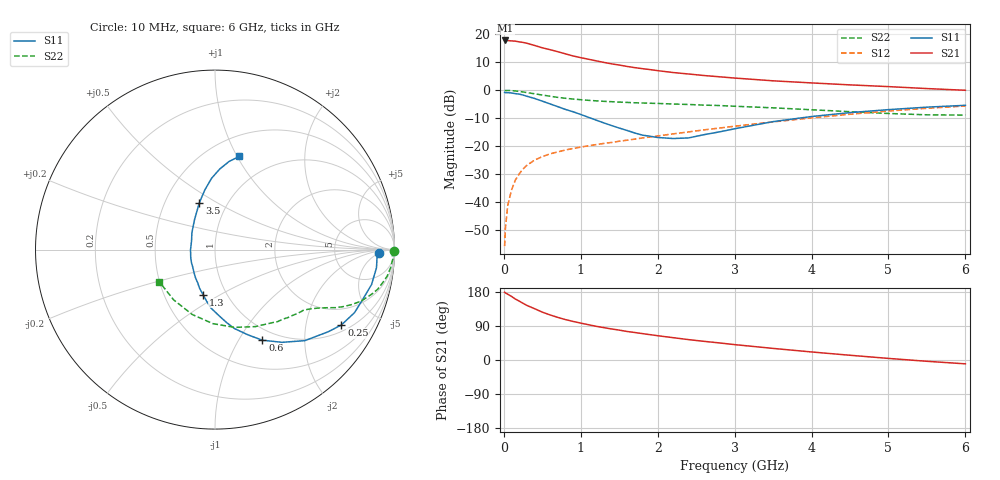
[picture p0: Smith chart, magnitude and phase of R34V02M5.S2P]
! SIEMENS Small Signal Semiconductors
! BFR181
! Si NPN RF Bipolar Junction Transistor in SOT23
! VCE = 4 V  IC = 2.5 mA
! Common Emitter S-Parameters:  May  1996
# GHz  S  MA  R  50
!  f  S11  S21  S12  S22
! GHz  MAG  ANG  MAG  ANG  MAG  ANG  MAG  ANG
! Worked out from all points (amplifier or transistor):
!   36 points, 10 MHz to 6 GHz, reference 50 ohm
!   highest |S21| = 17.9 dB at 20 MHz (marker M1)
!   |S21| within 3 dB of that: start of sweep to 554.5 MHz
!   unconditionally stable (mu >= 1): 1.491 GHz to 3.297 GHz
!   at 250 MHz: K = 0.26, MSG = 22.7 dB, |S12| = -28.2 dB
!   at 1.4 GHz: K = 0.98, MSG = 14.1 dB, |S12| = -18.7 dB
!   at 6 GHz: K = 0.86, MSG = 2.8 dB, |S12| = -5.6 dB
!   S11 on the Smith chart (normalised r, x): 10 MHz: 20, -5; 250 MHz: 1.24, -3.18; 600 MHz: 0.85, -1.27; 1.3 GHz: 0.78, -0.42; 3.5 GHz: 0.74, +0.41; 6 GHz: 0.70, +1.02
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0.01  0.9116 -1.3  7.794 178.8  0.0016 87.0  0.9963 -0.6
0.02  0.904 -2.4  7.815 177.2  0.0033 89.0  0.9865 -1.2
0.05  0.9054 -6.4  7.768 173.7  0.0085 87.3  0.9922 -3.0
0.1  0.8937 -12.6  7.68 167.8  0.0163 83.3  0.9841 -5.8
0.15  0.8686 -18.6  7.59 160.8  0.0245 78.3  0.9704 -8.8
0.25  0.8198 -30.8  7.203 149.5  0.0388 72.8  0.9329 -13.7
0.3  0.78 -35.9  6.963 144.0  0.0451 70.8  0.9088 -15.8
0.4  0.7125 -45.4  6.359 135.4  0.056 65.8  0.8636 -19.4
0.5  0.6377 -54.1  5.767 126.3  0.0645 62.4  0.8211 -21.9
0.6  0.5697 -62.4  5.344 119.0  0.0724 59.9  0.7812 -24.0
0.7  0.5089 -68.9  4.921 112.5  0.0783 58.3  0.7459 -25.7
0.8  0.4534 -76.1  4.496 106.7  0.0848 56.8  0.7179 -26.8
0.9  0.4114 -81.0  4.12 101.8  0.0904 56.4  0.6948 -27.8
1.1  0.3274 -93.7  3.598 93.1  0.1012 55.8  0.6597 -29.6
1.3  0.2598 -104.7  3.158 85.4  0.1114 56.1  0.6333 -31.2
1.6  0.1905 -124.9  2.676 75.3  0.1271 56.9  0.6052 -33.7
2.2  0.1363 -179.5  2.079 58.9  0.1652 58.0  0.5668 -40.3
2.6  0.1596 143.7  1.838 49.3  0.1945 57.6  0.5414 -45.7
3.5  0.2738 108.7  1.476 30.6  0.2707 53.5  0.4839 -62.5
4.5  0.3973 92.8  1.248 12.5  0.3716 44.9  0.4128 -91.6
5.5  0.4975 80.9  1.072 -3.4  0.4749 32.4  0.3626 -129.5
6  0.537 75.3  0.999 -10.1  0.5222 25.3  0.3584 -150.2
